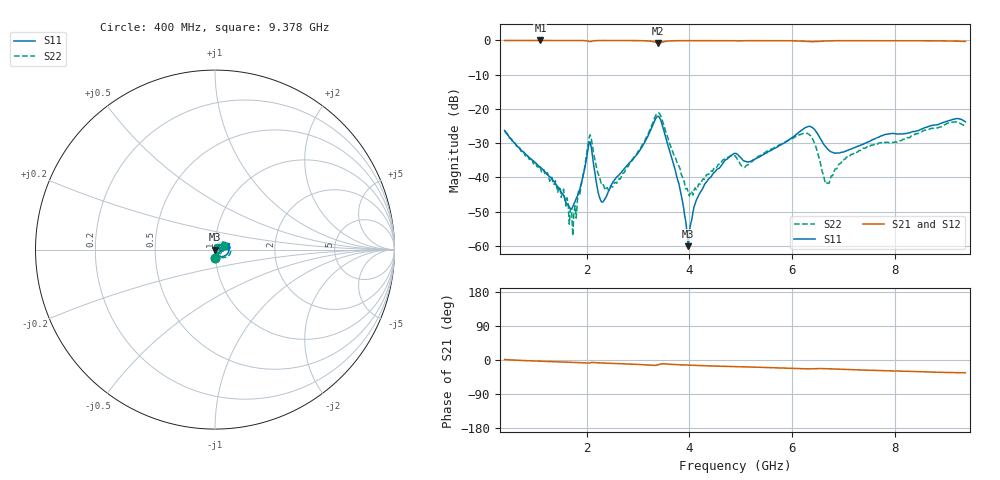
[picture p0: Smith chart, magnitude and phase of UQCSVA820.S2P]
!  Part Number  UQCSVA820  Mounting Orientation: Horizontal
!  Description: Ultra Low ESR Microwave capacitors
!  Application: Coupling, Bypass, Tuning, DC Block
!  Filters, Matching
# GHZ S DB R 50
! Freq  |S11|  S11 Ph  |S21|  S21 Ph  |S12|  S12 Ph  |S22|  S22 Ph
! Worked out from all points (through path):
!   400 points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, 400 MHz to 9.378 GHz, reference 50 ohm
!   highest |S21| = 0.00 dB at 1.098 GHz (marker M1); lowest = -0.7 dB at 3.393 GHz (marker M2)
!   group delay of S21, straight-line fit = 10.3 ps
!   lowest |S11| = -60.1 dB at 3.978 GHz (marker M3), VSWR 1.00, Z = 50.1 - j0.00585 ohm
!   |S11| at or under -10 dB: start of sweep to end of sweep
!   |S22| runs from -57.0 to -21.1 dB; largest |S21 - S12| = 0.0044
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0.4  -26.29 -87.9  -0.02 1.3  0.00 1.3  -26.50 -89.4
1.098  -37.05 -97.7  0.00 -3.2  -0.01 -3.2  -37.33 -96.8
1.548  -45.16 -130.4  -0.01 -5.3  -0.01 -5.3  -43.42 -80.2
1.638  -47.98 -147.2  -0.01 -5.7  -0.01 -5.8  -47.53 -83.1
1.66  -48.55 -156.3  -0.01 -5.8  -0.01 -5.9  -53.67 -62.0
1.705  -49.24 -168.8  -0.01 -6.1  -0.01 -6.1  -49.27 -54.6
1.728  -48.55 -177.9  -0.01 -6.2  -0.01 -6.2  -57.05 -38.0
1.75  -47.75 170.5  -0.01 -6.3  -0.01 -6.3  -50.21 11.3
1.795  -46.18 145.6  -0.01 -6.5  -0.01 -6.5  -51.88 7.6
1.908  -40.87 103.6  -0.02 -7.2  -0.01 -7.3  -40.90 41.2
2.065  -29.60 -1.6  -0.34 -7.3  -0.33 -7.3  -27.56 -13.5
2.313  -47.21 -176.7  -0.02 -8.0  -0.01 -8.1  -41.89 -38.9
2.65  -38.92 108.5  -0.02 -9.7  -0.01 -9.8  -40.53 24.5
3.393  -22.13 -1.4  -0.74 -12.4  -0.73 -12.5  -21.06 -6.1
3.798  -41.97 -81.8  -0.07 -12.6  -0.06 -12.7  -36.71 -57.5
3.978  -60.09 -3.4  -0.04 -13.6  -0.03 -13.7  -44.36 -28.8
4.18  -45.21 58.8  -0.03 -14.6  -0.02 -14.7  -41.95 33.0
4.9  -32.99 37.6  -0.11 -17.7  -0.10 -17.8  -33.86 37.9
6.408  -25.57 0.6  -0.35 -22.9  -0.36 -23.1  -29.01 9.6
6.655  -30.99 -10.6  -0.16 -22.9  -0.16 -23.1  -41.85 27.1
7.893  -27.26 37.1  -0.10 -28.5  -0.11 -28.6  -29.90 51.7
9.378  -23.76 17.7  -0.27 -33.5  -0.28 -33.7  -25.22 24.0
